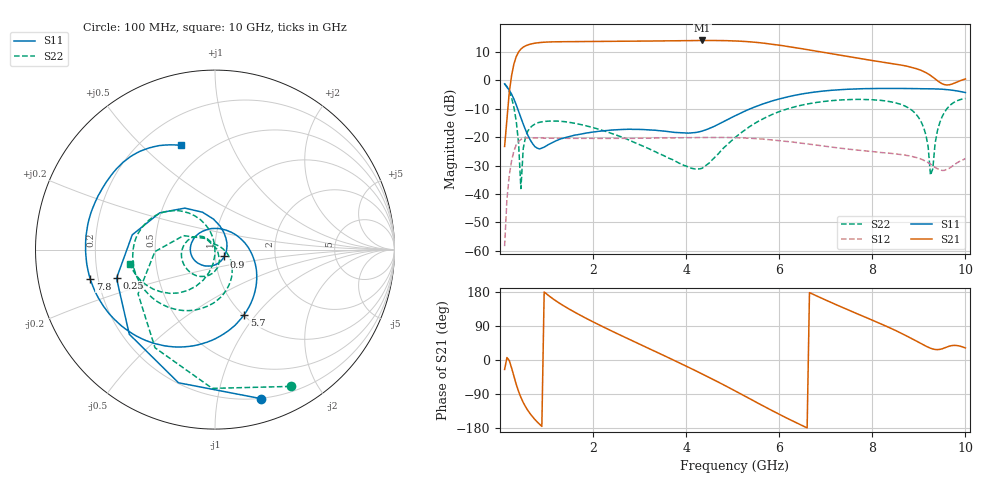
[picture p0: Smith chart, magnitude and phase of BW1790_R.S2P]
!Keysight Technologies,N5245A,MY52451660,A.10.49.11
!Date: Monday, August 07, 2017 16:38:14
!Correction: S11(Full 2 Port(1,2))
!S21(Full 2 Port(1,2))
!S12(Full 2 Port(1,2))
!S22(Full 2 Port(1,2))
!S2P File: Measurements: S11, S21, S12, S22:
# Hz S  dB  R 50
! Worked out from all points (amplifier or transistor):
!   199 points, 100 MHz to 10 GHz, reference 50 ohm
!   highest |S21| = 14.1 dB at 4.35 GHz (marker M1)
!   |S21| within 3 dB of that: 451.6 MHz to 6.519 GHz (6.067 GHz wide, 174 % of centre)
!   unconditionally stable (mu >= 1): start of sweep to end of sweep
!   at 1.75 GHz: K = 1.26, MAG = 14.0 dB, |S12| = -20.4 dB
!   at 5.05 GHz: K = 1.23, MAG = 14.2 dB, |S12| = -20.2 dB
!   at 10 GHz: K = 5.66, MAG = 3.5 dB, |S12| = -27.5 dB
!   S11 on the Smith chart (normalised r, x): 100 MHz: 0.20, -1.33; 250 MHz: 0.28, -0.13; 900 MHz: 1.11, -0.08; 5.7 GHz: 1.01, -0.87; 7.8 GHz: 0.17, -0.11; 10 GHz: 0.36, +0.66
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1e8  -1.23 -73.0  -23.27 -24.9  -58.40 -148.3  -1.20 -61.1
2.5e8  -4.86 -163.8  1.71 -20.9  -28.30 149.0  -6.12 -150.1
3.5e8  -8.63 146.4  8.38 -64.4  -22.69 103.8  -14.34 156.1
4.5e8  -13.16 108.5  11.05 -98.7  -20.80 70.1  -38.11 4.5
5e8  -15.39 92.8  11.72 -112.0  -20.43 57.7  -24.03 -65.8
7e8  -22.25 30.8  12.95 -149.7  -20.26 25.6  -15.92 -111.0
9e8  -23.82 -36.4  13.40 -175.2  -20.32 6.5  -14.60 -136.1
1.3e9  -20.62 -101.9  13.62 148.2  -20.39 -18.7  -14.41 -168.8
1.75e9  -18.85 -131.8  13.68 116.5  -20.42 -40.7  -15.62 165.2
2.5e9  -17.39 -166.2  13.76 70.7  -20.40 -71.5  -19.24 136.8
3.4e9  -17.68 146.0  13.90 18.9  -20.31 -106.1  -25.68 119.9
3.9e9  -18.50 104.7  14.00 -10.2  -20.18 -125.5  -29.43 104.5
4.35e9  -17.83 52.6  14.07 -37.2  -20.11 -143.6  -30.91 47.2
5.05e9  -12.48 -19.3  13.88 -81.4  -20.16 -173.6  -20.14 -31.6
5.7e9  -8.02 -65.9  13.04 -124.1  -20.75 157.4  -13.13 -70.8
6.15e9  -5.92 -92.0  12.04 -152.6  -21.47 138.6  -10.17 -95.3
6.7e9  -4.25 -120.2  10.58 175.0  -22.58 116.9  -8.04 -122.6
7.8e9  -2.92 -166.7  7.50 115.6  -24.75 80.3  -6.71 -171.0
8.35e9  -2.82 173.8  6.11 86.3  -25.62 61.9  -7.40 163.7
9.05e9  -2.94 149.9  3.53 43.2  -27.73 34.9  -14.61 116.0
9.25e9  -2.96 142.6  1.76 31.1  -29.49 29.2  -33.40 92.6
1e10  -4.28 108.2  0.51 31.7  -27.53 47.7  -6.37 -170.1
